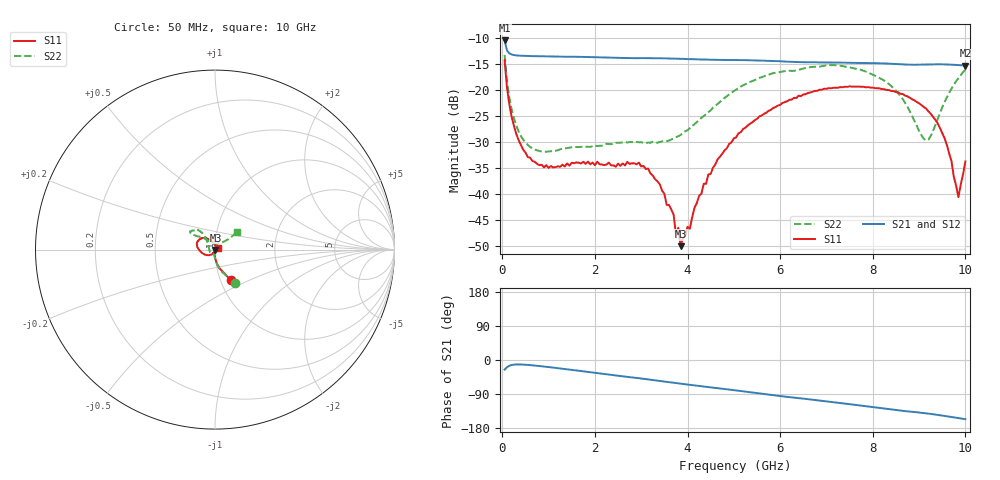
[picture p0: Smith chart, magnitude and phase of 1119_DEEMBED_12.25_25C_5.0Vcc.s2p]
!Hittite Microwave Corp.
!Digital Attenuator/PhaseShifter Rev 1.4.0
!Filename: C:\DATA\DATA\1119_DEEMBED_12.25_25C_5.0Vcc.s2p
!VNA ID: Agilent Technologies,N5224A,MY51441122,A.10.45.03
!Device type:
!2 Port Calibration.
!Temp(C): 25
!Lot Number:
!Serial Number:
!Operator:
!Misc:
!Attenuator:  12.250
# GHZ S DB R 50.0
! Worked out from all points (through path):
!   200 points, 50 MHz to 10 GHz, reference 50 ohm
!   highest |S21| = -10.54 dB at 50 MHz (marker M1); lowest = -15.4 dB at 10 GHz (marker M2)
!   group delay of S21, straight-line fit = 41.3 ps
!   lowest |S11| = -50.0 dB at 3.85 GHz (marker M3), VSWR 1.01, Z = 50.3 - j0.159 ohm
!   |S11| at or under -10 dB: start of sweep to end of sweep
!   |S22| runs from -31.9 to -13.3 dB; largest |S21 - S12| = 0.00054
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0.05  -14.36 -62.5  -10.54 -25.4  -10.54 -25.4  -13.32 -59.5
0.15  -22.70 -83.1  -13.00 -15.3  -13.00 -15.3  -21.44 -81.5
0.25  -26.90 -89.2  -13.34 -12.2  -13.34 -12.2  -25.45 -88.7
0.55  -32.93 -100.0  -13.53 -12.9  -13.52 -12.9  -30.59 -98.2
1  -35.02 -108.8  -13.60 -18.6  -13.60 -18.6  -31.85 -106.1
1.75  -33.83 -114.8  -13.70 -29.9  -13.70 -29.9  -30.91 -114.5
2.95  -33.99 -97.0  -13.93 -48.0  -13.94 -48.1  -30.09 -151.8
3.4  -38.13 -91.7  -13.96 -55.1  -13.97 -55.2  -30.05 -173.9
3.7  -44.00 -66.2  -14.02 -60.0  -14.02 -60.0  -29.37 169.3
3.75  -47.87 -59.2  -14.04 -60.8  -14.04 -60.9  -29.14 166.8
3.8  -46.52 -44.7  -14.05 -61.6  -14.05 -61.7  -28.92 163.0
3.85  -50.04 -30.3  -14.07 -62.4  -14.07 -62.5  -28.69 160.5
4.45  -36.25 73.9  -14.23 -71.5  -14.25 -71.6  -24.31 135.2
5.05  -29.14 100.2  -14.30 -80.3  -14.32 -80.3  -19.98 126.9
5.85  -23.51 122.2  -14.48 -92.9  -14.49 -93.0  -16.81 130.8
6.7  -20.38 138.4  -14.72 -104.8  -14.73 -104.8  -15.61 139.9
7.65  -19.37 158.8  -14.85 -118.8  -14.86 -118.8  -15.96 146.8
8.35  -20.06 171.8  -14.99 -129.6  -14.99 -129.7  -18.92 140.1
9.15  -23.61 -156.3  -15.15 -140.7  -15.17 -140.7  -29.72 89.6
9.55  -29.31 -125.1  -15.13 -147.6  -15.14 -147.6  -22.37 40.1
9.85  -40.62 -32.7  -15.27 -153.3  -15.27 -153.3  -17.76 38.2
10  -33.77 30.6  -15.37 -156.1  -15.38 -156.1  -16.15 39.3
